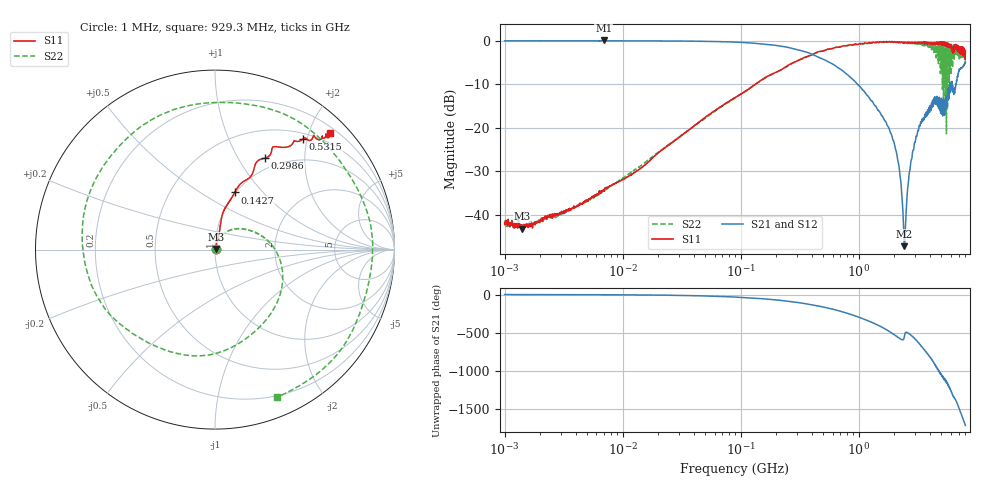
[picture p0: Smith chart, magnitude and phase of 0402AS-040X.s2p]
!s-Parameter Generated by FASTRON Sdn. Bhd.
!FASTRON P/N : 0402AS-040X
!Keysight Technologies: E5071C_MY46733604_B.14.02
!Date: Mon Dec 01 10:46:35 2025
!Version  :Rev00  Mon Dec 01 10:46:35 2025
!Data & Calibration Information:
!Freq  S11:SOLT2(ON)  S21:SOLT2(ON)  S12:SOLT2(ON)  S22:SOLT2(ON)
!PortZ  Port1:50+j0  Port2:50+j0
!When reading reference impedance value at option line is always used.
! Remarks : This data is being provided solely for informational purposes.
# Hz S dB R 50
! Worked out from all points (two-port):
!   1601 points, 1 MHz to 8 GHz, reference 50 ohm
!   highest |S21| = 0.01 dB at 6.912 MHz (marker M1); lowest = -47.2 dB at 2.428 GHz (marker M2)
!   |S21| within 3 dB of the highest: start of sweep to 388.4 MHz
!   lowest |S11| = -43.2 dB at 1.405 MHz (marker M3), VSWR 1.01, Z = 50.6 + j0.38 ohm
!   |S11| at or under -10 dB: start of sweep to 133.7 MHz
!   |S22| runs from -43.1 to -0.2 dB; largest |S21 - S12| = 0.022
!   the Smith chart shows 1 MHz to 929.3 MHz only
!   S11 on the Smith chart (normalised r, x): 1 MHz: 1.02, +0.01; 142.7 MHz: 0.99, +0.71; 298.6 MHz: 0.85, +1.30; 531.5 MHz: 0.60, +1.92; 929.3 MHz: 0.31, +2.35
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1000000  -41.80 23.3  -0.07 -0.4  -0.06 -0.4  -41.30 23.0
1404635  -43.20 32.9  -0.07 -0.5  -0.06 -0.5  -42.30 14.7
4479405  -37.40 60.0  -0.08 -1.7  -0.07 -1.7  -37.50 59.1
6911657  -34.50 61.0  0.01 -2.9  -0.16 -2.6  -34.20 59.9
2.00676e7  -25.70 75.0  -0.09 -7.6  -0.10 -7.5  -25.60 70.3
8.994653e7  -13.10 77.3  -0.37 -33.0  -0.37 -32.9  -13.10 29.1
1.426974e8  -9.45 70.9  -0.71 -51.5  -0.71 -51.5  -9.51 -0.0
2.986396e8  -4.74 61.5  -2.08 -103.0  -2.07 -103.0  -4.69 -91.1
4.006501e8  -3.32 56.6  -3.14 -135.0  -3.13 -135.0  -3.23 -149.0
5.3149e8  -2.10 51.5  -4.65 -173.0  -4.63 -173.0  -2.18 141.0
9.292726e8  -0.81 45.5  -9.40 80.5  -9.40 80.3  -0.99 -67.1
1.142645e9  -0.58 48.1  -12.10 28.4  -12.10 28.2  -0.70 -175.0
1.334081e9  -0.40 52.3  -14.50 -15.7  -14.50 -15.8  -0.56 91.7
1.542898e9  -0.33 58.1  -17.00 -62.3  -17.00 -62.4  -0.37 -7.6
1.7949e9  -0.25 64.4  -20.00 -119.0  -20.00 -120.0  -0.41 -129.0
2.082516e9  -0.33 71.1  -25.60 175.0  -25.60 175.0  -0.49 88.5
2.428208e9  -0.50 76.3  -47.20 161.0  -47.10 162.0  -0.36 -80.4
2.824359e9  -0.56 87.2  -26.80 176.0  -26.70 176.0  -0.34 93.2
3.183204e9  -0.42 96.9  -20.70 92.3  -20.70 91.9  -0.62 -91.3
3.548043e9  -0.43 108.0  -17.70 3.1  -17.70 2.8  -1.23 81.0
3.933151e9  -0.71 113.0  -15.30 -82.2  -15.30 -82.7  -1.56 -93.0
8e9  -2.28 -113.0  -5.01 84.9  -5.05 84.5  -4.70 120.0
